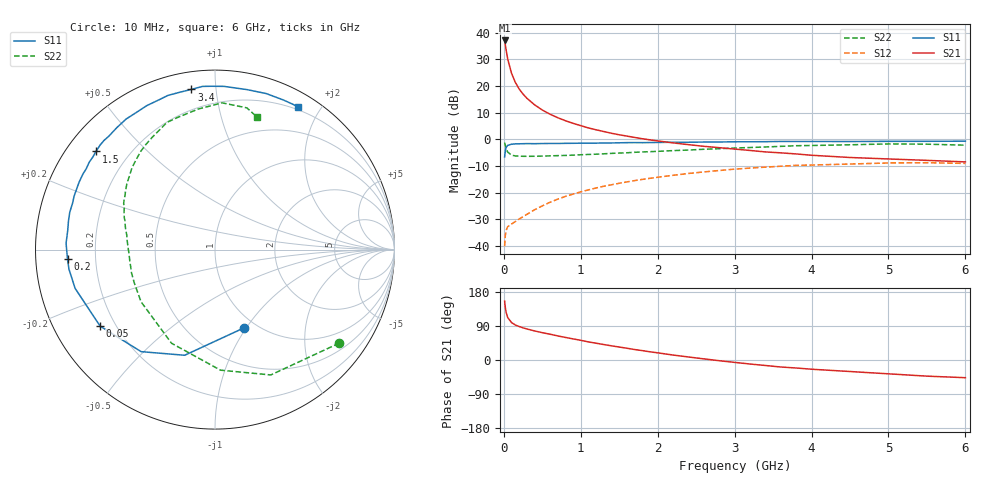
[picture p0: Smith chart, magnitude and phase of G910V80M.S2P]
! SIEMENS Small Signal Semiconductors
! BFG235
! Si NPN RF Bipolar Junction Transistor in SOT223
! VCE = 10 V  IC = 80 mA
! Common Emitter S-Parameters:  July  1994
# GHz  S  MA  R  50
!  f  S11  S21  S12  S22
! GHz  MAG  ANG  MAG  ANG  MAG  ANG  MAG  ANG
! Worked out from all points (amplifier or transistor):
!   40 points, 10 MHz to 6 GHz, reference 50 ohm
!   highest |S21| = 37.2 dB at 10 MHz (marker M1)
!   |S21| within 3 dB of that: start of sweep to 26.65 MHz
!   unconditionally stable (mu >= 1): 496.6 MHz to 1.437 GHz
!   at 200 MHz: K = 0.73, MSG = 24.4 dB, |S12| = -30.0 dB
!   at 1.5 GHz: K = 0.99, MSG = 9.1 dB, |S12| = -16.5 dB
!   at 6 GHz: K = 0.90, MSG = 0.3 dB, |S12| = -9.1 dB
!   S11 on the Smith chart (normalised r, x): 10 MHz: 0.87, -0.97; 50 MHz: 0.14, -0.30; 200 MHz: 0.10, -0.03; 1.5 GHz: 0.09, +0.36; 3.4 GHz: 0.09, +0.86; 6 GHz: 0.16, +1.73
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0.01  0.4652 -69.9  72.08 155.4  0.0098 68.0  0.8663 -37.0
0.02  0.6124 -106.0  58.83 137.5  0.0159 52.6  0.7644 -66.0
0.03  0.7019 -125.9  47.51 125.5  0.0193 43.3  0.6724 -87.4
0.05  0.769 -146.3  32.42 112.1  0.0228 34.5  0.5752 -114.9
0.1  0.8087 -164.5  17.37 98.8  0.0256 33.6  0.5043 -144.8
0.15  0.8208 -172.3  11.71 92.3  0.0285 38.5  0.4864 -157.6
0.2  0.8235 -176.3  8.784 88.2  0.0318 42.2  0.4829 -164.5
0.25  0.8264 -179.8  7.07 84.8  0.0351 46.2  0.4792 -169.0
0.3  0.8305 177.5  5.907 81.9  0.0389 49.8  0.4789 -172.6
0.4  0.8274 172.6  4.443 76.7  0.0474 53.3  0.4797 -177.3
0.5  0.832 168.8  3.549 72.1  0.0561 56.1  0.4837 179.1
0.6  0.8355 165.6  2.961 68.1  0.0655 57.2  0.4884 176.1
0.7  0.8347 161.9  2.549 63.6  0.075 58.0  0.4933 173.4
0.9  0.8413 156.6  1.996 55.7  0.0932 57.0  0.5039 168.9
1.1  0.8478 150.1  1.634 47.7  0.1122 55.3  0.519 164.6
1.5  0.8596 140.5  1.216 34.2  0.1491 49.8  0.5517 156.6
2.2  0.88 124.2  0.856 13.1  0.2106 38.0  0.6132 143.2
3.2  0.8983 102.6  0.617 -10.6  0.2874 18.6  0.7006 123.4
3.4  0.9022 98.4  0.579 -14.5  0.2996 14.5  0.7177 119.0
4.5  0.9091 78.6  0.455 -30.4  0.3428 -7.0  0.7886 96.8
5.5  0.9165 65.4  0.402 -42.6  0.363 -25.7  0.8093 77.3
6  0.9213 59.7  0.376 -46.7  0.3522 -32.5  0.7753 72.5
